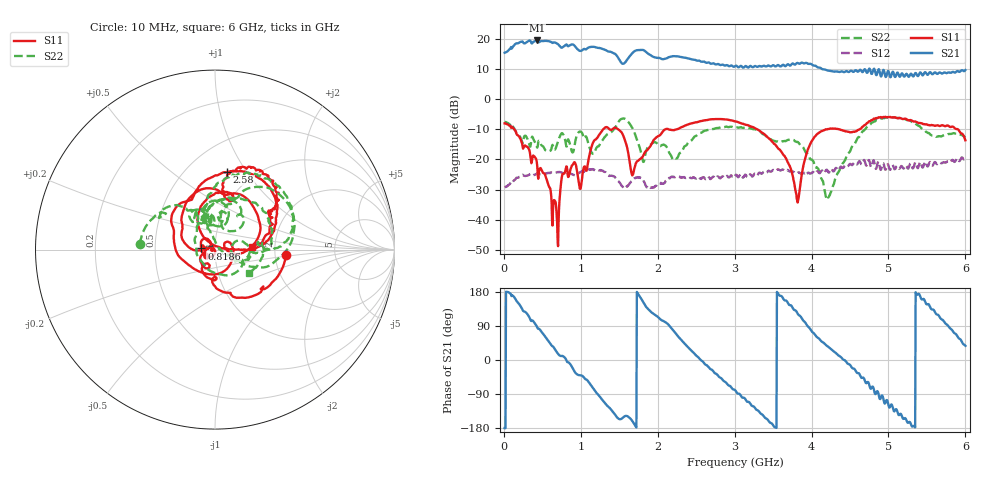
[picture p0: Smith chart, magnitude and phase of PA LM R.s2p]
!  29/10/2024  10:35:24
! Ref Plane: 0.000 mm
# MHZ S MA R  50
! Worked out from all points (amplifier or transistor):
!   1001 points, 10 MHz to 6 GHz, reference 50 ohm
!   highest |S21| = 19.5 dB at 429.3 MHz (marker M1)
!   |S21| within 3 dB of that: 69.84 MHz to 961.5 MHz (891.7 MHz wide, 173 % of centre)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
!   unconditionally stable (mu >= 1): start of sweep to 4.808 GHz; 4.809 GHz to 4.866 GHz; 4.938 GHz to end of sweep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
!   at 1.004 GHz: K = 1.36, MAG = 16.5 dB, |S12| = -24.1 dB
!   at 3.005 GHz: K = 2.00, MAG = 12.5 dB, |S12| = -25.5 dB
!   at 6 GHz: K = 1.58, MAG = 10.1 dB, |S12| = -19.5 dB
!   S11 on the Smith chart (normalised r, x): 10 MHz: 2.31, -0.15; 818.6 MHz: 0.86, +0.01; 2.58 GHz: 0.76, +0.82; 6 GHz: 1.52, +0.04
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10  0.3972 -4.0  5.898 -179.6  0.03454 0.8  0.4204 175.6
189.7  0.2475 -75.7  8.519 149.8  0.05016 -16.3  0.2611 122.8
429.3  0.08901 -154.4  9.427 88.2  0.05851 -61.9  0.1619 97.9
626.97  0.00974 135.0  8.628 36.8  0.06118 -100.3  0.1683 106.3
818.65  0.07617 175.4  8.042 -3.5  0.05578 -136.2  0.1642 81.8
926.47  0.08747 137.9  7.521 -32.9  0.05415 -152.6  0.1936 101.8
1010.33  0.04149 174.4  6.398 -40.9  0.06363 -164.8  0.2829 62.5
1231.96  0.2492 138.8  7.105 -92.8  0.066 144.0  0.1649 78.0
1417.65  0.3218 74.8  5.849 -137.1  0.05299 103.5  0.3036 68.1
1573.39  0.2088 5.9  4.021 -148.3  0.03384 90.2  0.4737 22.0
1723.14  0.08879 26.9  6.459 -178.2  0.05003 71.4  0.2268 -24.9
1842.94  0.1363 -82.8  6.149 141.8  0.03697 37.8  0.129 21.9
2010.66  0.2444 159.4  4.851 112.2  0.03976 37.0  0.1732 -17.2
2232.29  0.3126 113.5  5.154 70.6  0.05158 -3.3  0.1048 -166.3
2579.71  0.4376 81.3  4.185 -2.8  0.05043 -62.0  0.284 79.7
3005  0.4284 37.2  3.523 -79.4  0.05312 -129.8  0.3449 30.1
3544.1  0.1658 0.1  3.547 -179.2  0.06546 134.7  0.1987 -0.8
4005.33  0.2052 118.0  3.748 74.9  0.06077 53.2  0.09931 -28.8
4490.52  0.2859 72.1  2.845 -11.4  0.08296 -27.8  0.1311 108.8
5005.66  0.5034 54.9  2.784 -123.4  0.07516 -141.8  0.4968 46.5
5448.92  0.3864 35.1  2.501 161.1  0.07401 151.8  0.3174 -0.2
6000  0.2082 3.2  3.045 37.5  0.1061 42.7  0.2322 -34.3
